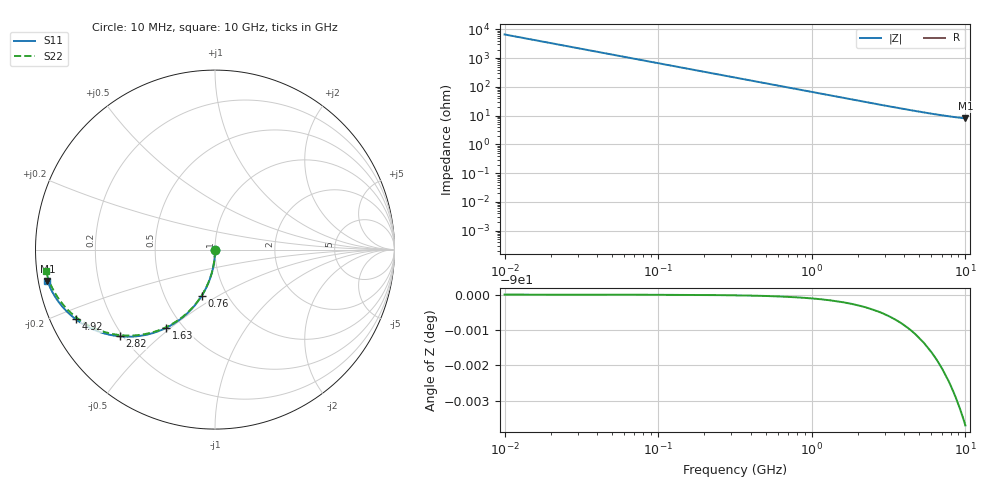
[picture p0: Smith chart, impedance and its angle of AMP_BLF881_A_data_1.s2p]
! Created Tue Feb 16 10:27:52 2010
# ghz S ma R 50
! 2 Port Network Data from SP1.SP block
! freq  magS11  angS11  magS21  angS21  magS12  angS12  magS22  angS22
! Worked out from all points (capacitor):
!   1000 points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, 10 MHz to 10 GHz, reference 50 ohm
!   read as one part in shunt: C = 2.39 pF near 60 MHz
!   lowest |Z| = 8.09 ohm at 10 GHz (marker M1)
!   S11 on the Smith chart (normalised r, x): 10 MHz: 1.00, -0.01; 760 MHz: 0.76, -0.42; 1.63 GHz: 0.41, -0.48; 2.82 GHz: 0.19, -0.38; 4.92 GHz: 0.07, -0.23; 10 GHz: 0.03, -0.09
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0.01  0.003684 -90.2  1 -0.2  1 -0.2  0.003684 -90.2
0.04  0.01473 -90.9  0.9999 -0.9  0.9999 -0.9  0.01473 -90.9
0.07  0.02578 -91.5  0.9997 -1.5  0.9997 -1.5  0.02578 -91.5
0.09  0.03314 -92.0  0.9994 -2.0  0.9994 -2.0  0.03314 -92.0
0.14  0.05151 -93.0  0.9987 -3.1  0.9987 -3.1  0.05151 -93.1
0.21  0.07714 -94.6  0.997 -4.6  0.997 -4.6  0.07714 -94.6
0.31  0.1135 -96.7  0.9935 -6.8  0.9935 -6.8  0.1135 -96.8
0.43  0.1565 -99.3  0.9877 -9.3  0.9877 -9.3  0.1565 -99.4
0.58  0.209 -102.4  0.9779 -12.5  0.9779 -12.5  0.209 -102.6
0.76  0.2697 -106.1  0.9629 -16.2  0.9629 -16.2  0.2697 -106.3
1.14  0.3872 -113.5  0.922 -23.7  0.922 -23.7  0.3871 -113.8
1.63  0.5143 -122.0  0.8576 -32.2  0.8576 -32.2  0.5143 -122.5
1.68  0.5257 -122.8  0.8507 -33.0  0.8507 -33.0  0.5257 -123.3
2.2  0.6281 -130.3  0.7781 -40.6  0.7781 -40.6  0.6281 -131.0
2.82  0.7176 -137.7  0.6965 -48.1  0.6965 -48.1  0.7176 -138.5
3.34  0.7719 -142.7  0.6357 -53.2  0.6357 -53.2  0.7719 -143.7
4.08  0.8267 -148.4  0.5626 -59.1  0.5626 -59.1  0.8267 -149.7
4.92  0.868 -153.5  0.4966 -64.3  0.4966 -64.3  0.868 -155.0
5.01  0.8715 -154.0  0.4904 -64.8  0.4904 -64.8  0.8715 -155.5
6.67  0.9156 -160.9  0.402 -72.0  0.402 -72.0  0.9156 -163.0
8.34  0.9379 -165.7  0.3469 -77.1  0.3469 -77.1  0.9378 -168.5
10  0.9496 -169.4  0.3132 -81.1  0.3132 -81.1  0.9496 -172.8
